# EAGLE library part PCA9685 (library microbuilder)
PCA9685 - 16 Channel 12-Bit I2C PWM Controller 5.0V tolerant 16 channel, 12-bit I2C PWM controller with 25mA per output (max. 400mA total) Digikey: 568-5931-1-ND
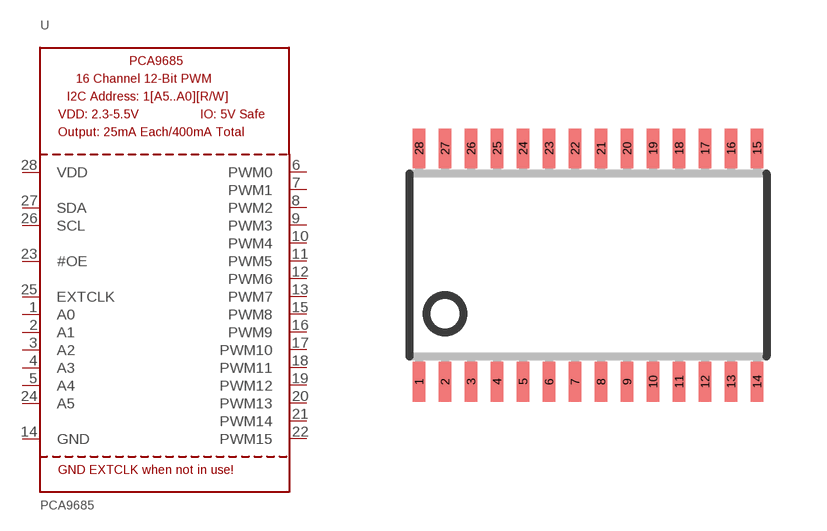
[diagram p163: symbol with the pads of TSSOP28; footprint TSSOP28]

Designator prefix U

## PCA9685  [TSSOP28]
1  A0
2  A1
3  A2
4  A3
5  A4
6  PWM0  out
7  PWM1  out
8  PWM2  out
9  PWM3  out
10  PWM4  out
11  PWM5  out
12  PWM6  out
13  PWM7  out
14  GND  pwr
15  PWM8  out
16  PWM9  out
17  PWM10  out
18  PWM11  out
19  PWM12  out
20  PWM13  out
21  PWM14  out
22  PWM15  out
23  #OE  in
24  A5
25  EXTCLK  in
26  SCL
27  SDA
28  VDD  pwr

## Footprint TSSOP28 (pad centres in mm)
smd 0.305 x 0.991: 1 -4.225,-2.918; 2 -3.575,-2.918; 3 -2.925,-2.918; 4 -2.275,-2.918; 5 -1.625,-2.918; 6 -0.975,-2.918; 7 -0.325,-2.918; 8 0.325,-2.918; 9 0.975,-2.918; 10 1.625,-2.918; 11 2.275,-2.918; 12 2.925,-2.918; 13 3.575,-2.918; 14 4.225,-2.918; 15 4.225,2.918; 16 3.575,2.918; 17 2.925,2.918; 18 2.275,2.918; 19 1.625,2.918; 20 0.975,2.918; 21 0.325,2.918; 22 -0.325,2.918; 23 -0.975,2.918; 24 -1.625,2.918; 25 -2.275,2.918; 26 -2.925,2.918; 27 -3.575,2.918; 28 -4.225,2.918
